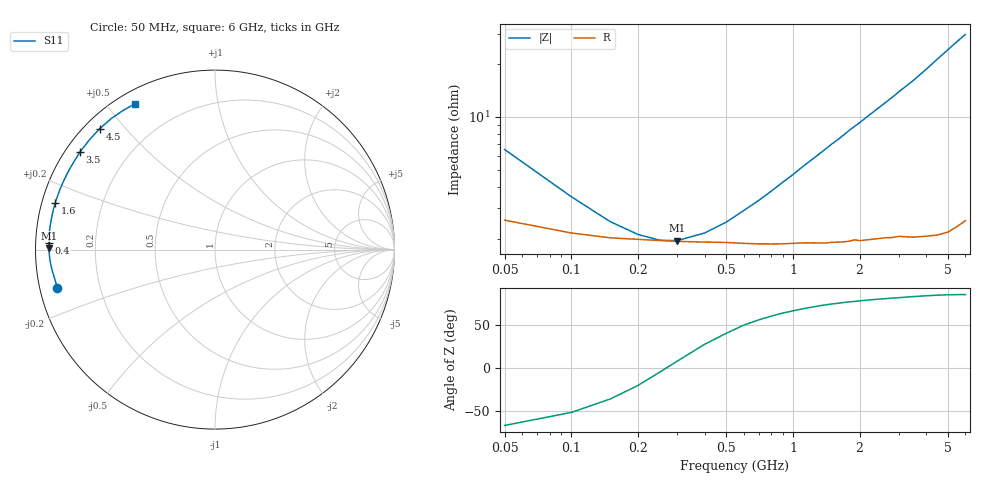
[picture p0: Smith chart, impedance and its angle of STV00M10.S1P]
! SIEMENS Discrete & RF Semiconductors
! BA892
! Si PIN Diode in SCD-80
! IF = 0.1 mA
! S-Parameters:  September  1997
# GHz  S  MA  R  50
!  f  S11
! GHz  MAG  ANG
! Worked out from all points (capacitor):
!   34 points, 50 MHz to 6 GHz, reference 50 ohm
!   read as one part to ground: C = 500 pF near 50 MHz
!   lowest |Z| = 1.96 ohm at 300 MHz (marker M1)
!   series resonance near 270 MHz, so ESL is about 690 pH
!   S11 on the Smith chart (normalised r, x): 50 MHz: 0.05, -0.12; 400 MHz: 0.04, +0.02; 1.6 GHz: 0.04, +0.14; 3.5 GHz: 0.04, +0.32; 4.5 GHz: 0.04, +0.43; 6 GHz: 0.05, +0.59
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0.05  0.9035 -166.3
0.1  0.917 -173.7
0.15  0.9217 -176.6
0.2  0.9232 -178.3
0.25  0.9243 -179.6
0.3  0.9251 179.4
0.4  0.9258 177.7
0.6  0.9271 174.9
0.8  0.9278 172.5
0.9  0.9278 171.3
1  0.9275 170.2
1.1  0.9272 169.0
1.4  0.9277 165.7
1.5  0.9273 164.6
1.6  0.9273 163.6
1.8  0.9267 161.4
1.9  0.9258 160.4
2  0.9267 159.4
2.2  0.9263 157.3
2.4  0.926 155.3
2.8  0.9261 151.3
3  0.9256 149.2
3.5  0.9282 144.3
4  0.9295 139.0
4.5  0.9309 133.6
5  0.9312 128.4
5.5  0.9292 123.4
6  0.927 118.8
